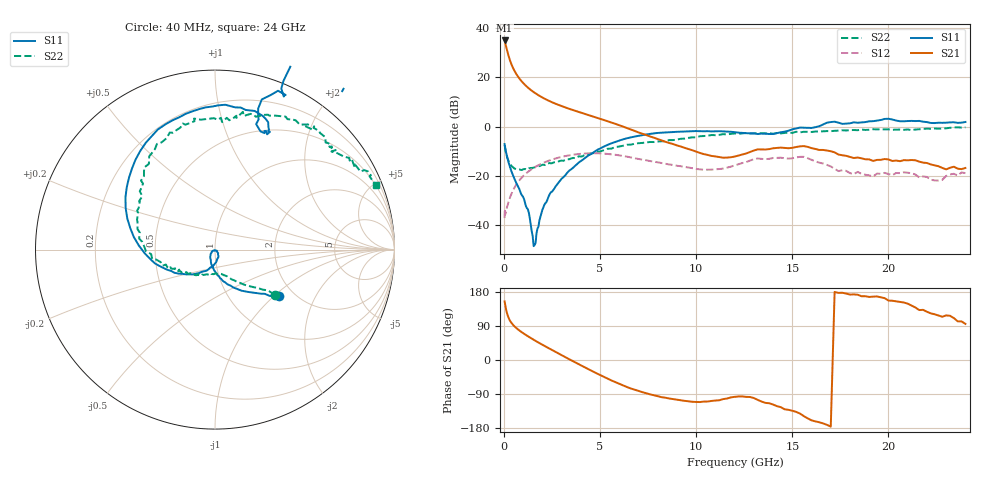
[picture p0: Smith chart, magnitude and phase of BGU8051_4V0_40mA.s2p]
! BGU8051_4V0_40mA
! Date/time Tue Jun 16 11:03:17 2015
! VAR V_out= 4.0000
! VAR I_out= 39.9800
! VAR V_in= 4.6600
! VAR I_in= 0.5426
# MHz S MA R 50
!  Freq-MHz  S11-mag  S11-arg  S21-mag  S21-arg  S12-mag  S12-arg  S22-mag  S22-arg
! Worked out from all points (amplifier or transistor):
!   187 points, 40 MHz to 24 GHz, reference 50 ohm
!   highest |S21| = 34.9 dB at 40 MHz (marker M1)
!   |S21| within 3 dB of that: start of sweep to 137 MHz
!   unconditionally stable (mu >= 1): 490.4 MHz to 13.36 GHz; 13.42 GHz to 14.03 GHz
!   at 750 MHz: K = 1.01, MAG = 20.5 dB, |S12| = -22.4 dB
!   at 5.4 GHz: K = 1.20, MAG = 3.9 dB, |S12| = -11.1 dB
!   at 24 GHz: K = -0.49, MSG = 1.0 dB, |S12| = -18.9 dB
!   lowest NFmin = 0.34 dB at 400 MHz
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40  0.44 -35.9  55.59 154.7  0.01391 31.0  0.4189 -37.4
50  0.4097 -35.2  53.7 152.4  0.02134 74.2  0.3965 -37.3
60  0.4025 -40.1  52.3 149.0  0.02128 42.4  0.3735 -37.6
80  0.3562 -43.7  48.29 143.2  0.01696 39.3  0.3311 -41.1
120  0.298 -52.2  41.84 132.6  0.0197 45.8  0.2821 -46.4
160  0.2545 -60.1  36.07 124.2  0.02253 48.8  0.2485 -51.0
200  0.2194 -66.5  31.32 117.5  0.0255 52.1  0.2221 -55.1
220  0.2052 -70.3  29.39 114.6  0.02772 54.0  0.2134 -56.3
280  0.1694 -77.6  24.44 107.5  0.03275 56.5  0.1888 -61.1
360  0.1349 -86.5  19.82 100.5  0.03989 59.4  0.1653 -65.2
440  0.11 -93.7  16.59 95.0  0.04734 60.4  0.1531 -70.2
550  0.08706 -102.4  13.54 88.9  0.05747 60.7  0.1408 -74.9
700  0.06552 -110.9  10.78 82.1  0.07123 59.7  0.1355 -80.3
950  0.04015 -129.1  8.046 72.6  0.09381 56.3  0.1323 -89.9
1550  0.003749 -134.7  4.989 53.4  0.145 45.1  0.1466 -109.8
2600  0.05331 -75.9  2.993 23.7  0.2198 22.4  0.1876 -132.7
4100  0.2114 -139.1  1.861 -16.5  0.2817 -11.3  0.25 -154.7
8200  0.7507 111.5  0.5237 -98.1  0.1816 -76.2  0.5013 147.5
12200  0.7515 66.7  0.2582 -96.2  0.1721 -73.5  0.7151 103.3
16200  0.9701 67.6  0.3508 -162.0  0.1968 -149.5  0.7915 70.7
20200  1.389 33.7  0.2003 156.4  0.1032 -155.4  0.8576 44.0
24000  1.236 20.9  0.1444 95.2  0.1135 -172.3  0.9657 21.8
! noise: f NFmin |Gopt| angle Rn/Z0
400  0.3394  0.06965  7.87  0.0486
550  0.3447  0.04796  29.37  0.0486
950  0.3716  0.05296  116  0.0481
1250  0.4037  0.08478  140.2  0.0475
1600  0.4542  0.1189  154.6  0.047
1900  0.5086  0.144  163.8  0.0469
2250  0.5851  0.1697  173.4  0.0478
2600  0.6756  0.1936  182.4  0.0501
3300  0.8985  0.242  198.8  0.0608
4000  1.177  0.2951  212  0.0826
